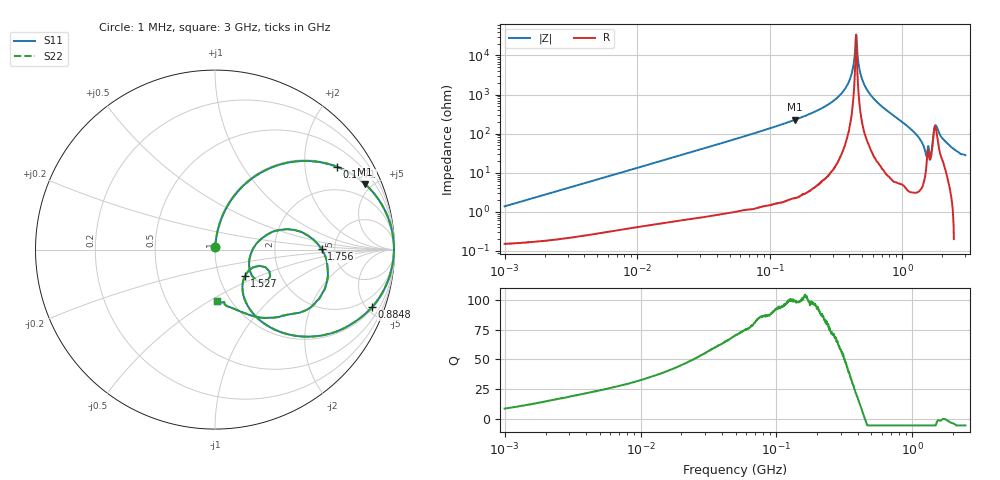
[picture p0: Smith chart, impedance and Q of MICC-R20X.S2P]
!s-Parameter Generated by FASTRON Sdn. Bhd.
!FASTRON P/N : MICC-R20X
!Keysight Technologies,E4991B,MY54100416,A.01.15
!Date: Wed Aug 26 13:53:51 2026
!Version  : Rev00 Wed Aug 26 13:53:51 2026
!Data & Calibration Information:
!PortZ  Port1:50+j0  Port2:50+j0
!When reading, reference impedance value at option line is always used.
! Remarks : This data is being provided solely for informational purposes.
!Freq	S11	S21	S12	S22
# Hz S dB R 50
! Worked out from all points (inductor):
!   1601 points, 1 MHz to 3 GHz, reference 50 ohm
!   read as one part in series: L = 218 nH near 1.041 MHz
!   highest Q = 101 at 155.9 MHz (marker M1), where L = 232 nH
!   self-resonance near 448 MHz
!   S11 on the Smith chart (normalised r, x): 1 MHz: 1.00, +0.03; 107.1 MHz: 1.03, +2.94; 884.8 MHz: 1.12, -5.40; 1.527 GHz: 1.32, -0.41; 1.756 GHz: 3.93, +0.03; 3 GHz: 0.86, -0.54
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1000000  -37.21 82.9  -0.01 -0.8  -0.01 -0.8  -37.21 82.9
3804036  -25.82 84.4  -0.03 -2.9  -0.03 -2.9  -25.82 84.4
1.447069e7  -14.56 77.8  -0.20 -10.8  -0.20 -10.8  -14.56 77.8
5.477226e7  -4.69 53.6  -1.89 -35.6  -1.89 -35.6  -4.69 53.6
1.070951e8  -1.70 34.1  -5.03 -55.3  -5.03 -55.3  -1.70 34.1
1.558689e8  -0.80 23.6  -7.94 -65.8  -7.94 -65.8  -0.80 23.6
2.083556e8  -0.39 16.5  -10.95 -72.9  -10.95 -72.9  -0.39 16.5
3.631036e8  -0.05 4.5  -22.13 -83.6  -22.13 -83.6  -0.05 4.5
4.073935e8  -0.03 2.1  -28.72 -83.8  -28.72 -83.8  -0.03 2.1
4.369573e8  -0.02 0.6  -39.33 -75.1  -39.33 -75.1  -0.02 0.6
4.502753e8  -0.02 -0.0  -50.78 14.1  -50.78 14.1  -0.02 -0.0
4.616833e8  -0.02 -0.6  -39.42 74.2  -39.42 74.2  -0.02 -0.6
4.902556e8  -0.03 -1.9  -29.45 82.9  -29.45 82.9  -0.03 -1.9
5.311214e8  -0.05 -3.8  -23.64 83.1  -23.64 83.1  -0.05 -3.8
7.925923e8  -0.38 -15.5  -11.46 73.2  -11.46 73.2  -0.38 -15.5
8.848309e8  -0.62 -20.2  -9.25 68.6  -9.25 68.6  -0.62 -20.2
1.287806e9  -3.52 -46.3  -2.81 41.8  -2.81 41.8  -3.52 -46.3
1.526649e9  -13.04 -41.9  -1.44 10.1  -1.44 10.1  -13.04 -41.9
1.653904e9  -13.47 1.6  -2.07 -0.4  -2.07 -0.4  -13.47 1.6
1.75626e9  -4.51 0.2  -7.84 -0.3  -7.84 -0.3  -4.51 0.2
1.980367e9  -5.16 -40.6  -3.31 31.7  -3.31 31.7  -5.16 -40.6
3e9  -10.79 -87.7  0.25 16.3  0.25 16.3  -10.79 -87.7
